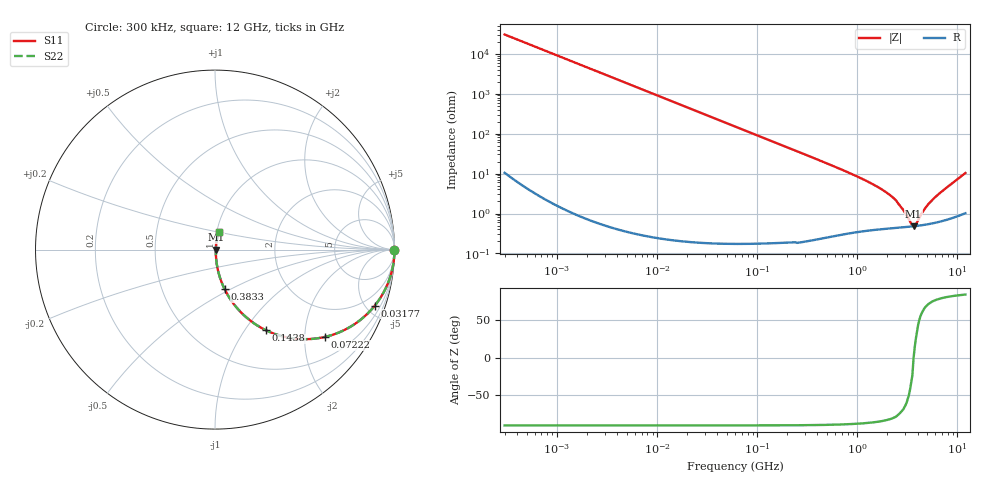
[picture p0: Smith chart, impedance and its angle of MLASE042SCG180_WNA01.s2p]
! MLASE042SCG180_WNA01  S-PARAMETER MODEL  ( General Type )
! Model Generated by TAIYO YUDEN Corporation (http://www.ty-top.com)
! Version 1.0
! TAIYO YUDEN Control No. 130801
! Copyright(c) 2013 TAIYO YUDEN CO.,LTD. All Rights Reserved.
! Product Description (link to TY-COMPAS)
! https://ds.yuden.co.jp/TYCOMPAS/or/detail?pn=MLASE042SCG180JWNA01&u=M
! Products Name : Multilayer Ceramic Capacitors
! Characteristics :
!  Capacitance : 18 pF , Rated Voltage : 16V , TCC : CG / C0G
!  Case Size : 0.4 x 0.2 / 0.016 x 0.008 [mm/inch] , Thickness : 0.2 / 0.008 [mm/inch]
!  (Conditions: Temperature = 25 degC , DC Bias Current/Voltage = 0A / 0V)
! External Node Assignments :
!  1  o---| |---o  2
! GND o---------o GND
! Frequency Range : 0.3MHz  -  12000MHz  [ 401 STEP ]
# MHz S RI R 50
! Freq[MHz].  S11 Real  S11 Imag  S21 Real  S21 Imag  S12 Real  S12 Imag  S22 Real  S22 Imag
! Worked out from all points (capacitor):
!   401 points, 300 kHz to 12 GHz, reference 50 ohm
!   read as one part in series: C = 17.5 pF near 316.3 kHz
!   lowest |Z| = 478 mohm at 3.643 GHz (marker M1)
!   series resonance near 3.646 GHz, so ESL is about 110 pH
!   S11 on the Smith chart (normalised r, x): 300 kHz: open; 31.77 MHz: 1.00, -5.72; 72.22 MHz: 1.00, -2.51; 143.8 MHz: 1.00, -1.26; 383.3 MHz: 1.00, -0.47; 12 GHz: 1.02, +0.21
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0.3  1 -0.0033  1.2e-05 0.0033  1.2e-05 0.0033  1 -0.0033
1.769972  0.9996 -0.0195  0.000383 0.0195  0.000383 0.0195  0.9996 -0.0195
10.44266  0.9869 -0.1134  0.0131 0.1134  0.0131 0.1134  0.9869 -0.1134
19.72127  0.9549 -0.2073  0.0451 0.2073  0.0451 0.2073  0.9549 -0.2073
31.77076  0.8909 -0.3115  0.1091 0.3115  0.1091 0.3115  0.8909 -0.3115
60  0.696 -0.4594  0.304 0.4594  0.304 0.4594  0.696 -0.4594
72.22496  0.6124 -0.4865  0.3876 0.4865  0.3876 0.4865  0.6124 -0.4865
101.9188  0.4425 -0.4957  0.5575 0.4957  0.5575 0.4957  0.4425 -0.4957
143.8206  0.2851 -0.4501  0.7149 0.4501  0.7149 0.4501  0.2851 -0.4501
219.7372  0.1462 -0.3511  0.8538 0.3511  0.8538 0.3511  0.1462 -0.3511
353.9943  0.0625 -0.2379  0.9375 0.2379  0.9375 0.2379  0.0625 -0.2379
383.2761  0.054 -0.2213  0.946 0.2213  0.946 0.2213  0.054 -0.2213
1135.593  0.00872 -0.0714  0.9913 0.0714  0.9913 0.0714  0.00872 -0.0714
2088.533  0.00505 -0.0291  0.995 0.0291  0.995 0.0291  0.00505 -0.0291
2514.07  0.0047 -0.0183  0.9953 0.0183  0.9953 0.0183  0.0047 -0.0183
2947.191  0.00461 -0.01  0.9954 0.01  0.9954 0.01  0.00461 -0.01
3454.93  0.0047 -0.00293  0.9953 0.00293  0.9953 0.00293  0.0047 -0.00293
3642.919  0.00476 -4.12e-05  0.9952 4.12e-05  0.9952 4.12e-05  0.00476 -4.12e-05
3841.137  0.00484 0.00231  0.9952 -0.00231  0.9952 -0.00231  0.00484 0.00231
4747.894  0.00536 0.0123  0.9946 -0.0123  0.9946 -0.0123  0.00536 0.0123
5715.274  0.00616 0.022  0.9938 -0.022  0.9938 -0.022  0.00616 0.022
12000  0.0202 0.0999  0.9798 -0.0999  0.9798 -0.0999  0.0202 0.0999
